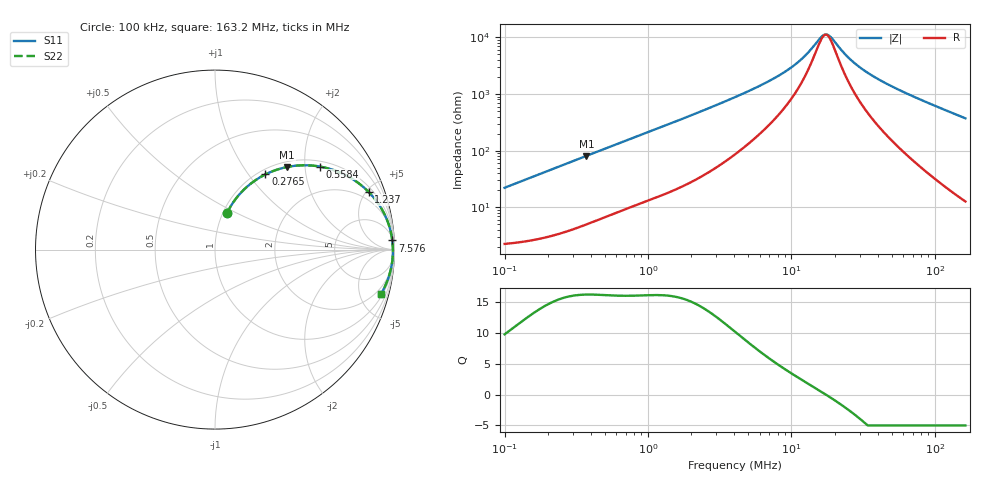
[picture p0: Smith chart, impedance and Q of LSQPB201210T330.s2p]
! LSQPB201210T330  S-PARAMETER MODEL  ( General Type )
! Model Generated by TAIYO YUDEN Corporation (http://www.ty-top.com)
! Version 2.0
! TAIYO YUDEN Control No. 100810NF18SB-HKC
! Copyright(c) 2007 TAIYO YUDEN CO.,LTD. All Rights Reserved.
! Product Description (link to TY-COMPAS)
! https://ds.yuden.co.jp/TYCOMPAS/or/detail?pn=LSQPB201210T330M&u=M
! Products Name : Inductors
! Characteristics :
!  Inductance : 33 uH , SRF(min) : 8.0 MHz , DC Resistance(max) : 2.6 Ohm
!  Rated Current : Saturation :150 mA , Temp Rise : 220 mA (40 degC)
!  Case Size : 2.0 x 1.25 / 0.079 x 0.049 [mm/inch] , Thickness : 1.0 / 0.04 [mm/inch]
!  (Conditions: Temperature = 25 degC , DC Bias Current/Voltage = 0A / 0V)
! External Node Assignments :
!  1  o---GGG---o  2
! GND o---------o GND
! Frequency Range : 0.1MHz  -  163.203978MHz  [ 402 STEP ]
# MHz S RI R 50
! Freq[MHz].  S11 Real  S11 Imag  S21 Real  S21 Imag  S12 Real  S12 Imag  S22 Real  S22 Imag
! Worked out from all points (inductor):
!   401 points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, 100 kHz to 163.2 MHz, reference 50 ohm
!   read as one part in series: L = 35.1 uH near 103.8 kHz
!   highest Q = 16.2 at 371.8 kHz (marker M1), where L = 34.6 uH
!   self-resonance near 17.09 MHz
!   S11 on the Smith chart (normalised r, x): 100 kHz: 1.05, +0.44; 276.5 kHz: 1.08, +1.21; 558.4 kHz: 1.15, +2.40; 1.237 MHz: 1.32, +5.20; 7.576 MHz: 8, +37; 163.2 MHz: 1.25, -7.44
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0.1  0.0657 0.2017  0.9343 -0.2017  0.9343 -0.2017  0.0657 0.2017
0.170971  0.142 0.3144  0.858 -0.3144  0.858 -0.3144  0.142 0.3144
0.276535  0.2812 0.4191  0.7188 -0.4191  0.7188 -0.4191  0.2812 0.4191
0.345249  0.3701 0.4528  0.6299 -0.4528  0.6299 -0.4528  0.3701 0.4528
0.371757  0.4022 0.4604  0.5978 -0.4604  0.5978 -0.4604  0.4022 0.4604
0.558419  0.586 0.4623  0.414 -0.4623  0.414 -0.4623  0.586 0.4623
0.823433  0.7411 0.4079  0.2589 -0.4079  0.2589 -0.4079  0.7411 0.4079
1.191969  0.8483 0.329  0.1517 -0.329  0.1517 -0.329  0.8483 0.329
1.236883  0.8567 0.3206  0.1433 -0.3206  0.1433 -0.3206  0.8567 0.3206
2.075963  0.9374 0.2109  0.0626 -0.2109  0.0626 -0.2109  0.9374 0.2109
4.115259  0.9773 0.1073  0.0227 -0.1073  0.0227 -0.1073  0.9773 0.1073
7.576131  0.9876 0.0508  0.0124 -0.0508  0.0124 -0.0508  0.9876 0.0508
10.76595  0.9899 0.0273  0.0101 -0.0273  0.0101 -0.0273  0.9899 0.0273
13.94754  0.9908 0.0122  0.00923 -0.0122  0.00923 -0.0122  0.9908 0.0122
16.47344  0.9911 0.00286  0.00891 -0.00286  0.00891 -0.00286  0.9911 0.00286
18.06938  0.9912 -0.00228  0.00881 0.00228  0.00881 0.00228  0.9912 -0.00228
23.84629  0.9911 -0.0181  0.00886 0.0181  0.00886 0.0181  0.9911 -0.0181
28.16483  0.9908 -0.0283  0.00918 0.0283  0.00918 0.0283  0.9908 -0.0283
35.81962  0.9898 -0.0444  0.0102 0.0444  0.0102 0.0444  0.9898 -0.0444
48.15376  0.9873 -0.0679  0.0127 0.0679  0.0127 0.0679  0.9873 -0.0679
85.43126  0.9741 -0.1315  0.0259 0.1315  0.0259 0.1315  0.9741 -0.1315
163.204  0.9254 -0.2462  0.0746 0.2462  0.0746 0.2462  0.9254 -0.2462
